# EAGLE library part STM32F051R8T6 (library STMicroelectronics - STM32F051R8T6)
Source: Datasheet
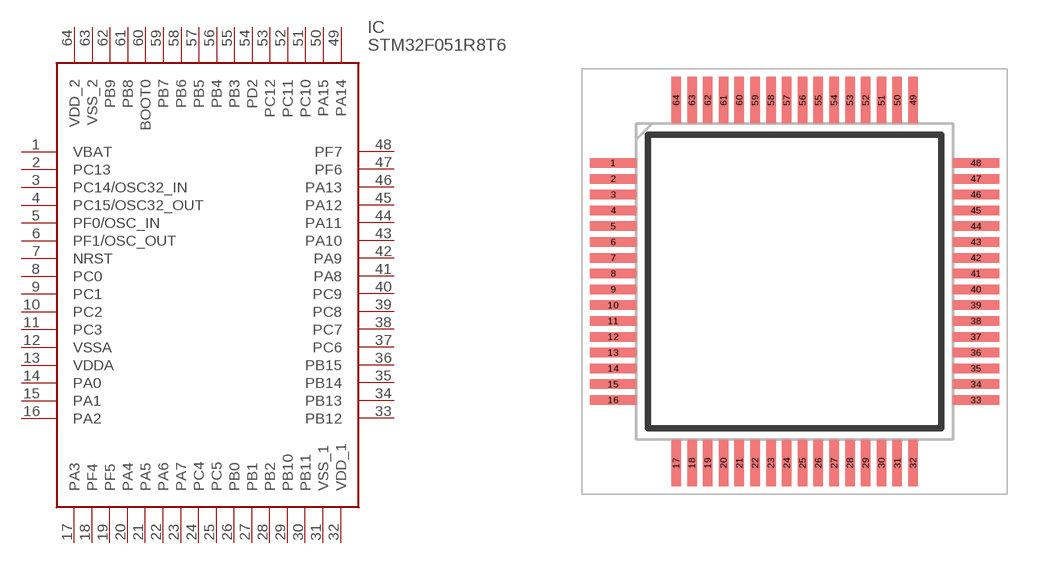
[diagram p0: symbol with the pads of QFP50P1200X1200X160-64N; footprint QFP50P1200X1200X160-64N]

Designator prefix IC

## STM32F051R8T6 (ALLIED_NUMBER: 70390941; ALLIED_PRICE-STOCK: http://www.alliedelec.com/stmicroelectronics-stm32f051r8t6/70390941/; HEIGHT: 1.6mm; MANUFACTURER_NAME: STMicroelectronics; MANUFACTURER_PART_NUMBER: STM32F051R8T6; MOUSER_PART_NUMBER: 511-STM32F051R8T6; MOUSER_PRICE-STOCK: https://www.mouser.com/Search/Refine.aspx?Keyword=511-STM32F051R8T6; RS_PART_NUMBER: 7618683P; RS_PRICE-STOCK: http://uk.rs-online.com/web/p/products/7618683P)  [QFP50P1200X1200X160-64N]
1  VBAT
2  PC13
3  PC14/OSC32_IN  in
4  PC15/OSC32_OUT  out
5  PF0/OSC_IN  in
6  PF1/OSC_OUT  out
7  NRST  in
8  PC0
9  PC1
10  PC2
11  PC3
12  VSSA  pwr
13  VDDA  pwr
14  PA0
15  PA1
16  PA2
17  PA3
18  PF4
19  PF5
20  PA4
21  PA5
22  PA6
23  PA7
24  PC4
25  PC5
26  PB0
27  PB1
28  PB2
29  PB10
30  PB11
31  VSS_1  pwr
32  VDD_1  pwr
33  PB12
34  PB13
35  PB14
36  PB15
37  PC6
38  PC7
39  PC8
40  PC9
41  PA8
42  PA9
43  PA10
44  PA11
45  PA12
46  PA13
47  PF6
48  PF7
49  PA14
50  PA15
51  PC10
52  PC11
53  PC12
54  PD2
55  PB3
56  PB4
57  PB5
58  PB6
59  PB7
60  BOOT0
61  PB8
62  PB9
63  VSS_2  pwr
64  VDD_2  pwr

## Footprint QFP50P1200X1200X160-64N (pad centres in mm)
LQFP64-10 x 10 mm 64 pin
smd 1.475 x 0.3: 1 -5.738,3.75; 2 -5.738,3.25; 3 -5.738,2.75; 4 -5.738,2.25; 5 -5.738,1.75; 6 -5.738,1.25; 7 -5.738,0.75; 8 -5.738,0.25; 9 -5.738,-0.25; 10 -5.738,-0.75; 11 -5.738,-1.25; 12 -5.738,-1.75; 13 -5.738,-2.25; 14 -5.738,-2.75; 15 -5.738,-3.25; 16 -5.738,-3.75; 33 5.738,-3.75; 34 5.738,-3.25; 35 5.738,-2.75; 36 5.738,-2.25; 37 5.738,-1.75; 38 5.738,-1.25; 39 5.738,-0.75; 40 5.738,-0.25; 41 5.738,0.25; 42 5.738,0.75; 43 5.738,1.25; 44 5.738,1.75; 45 5.738,2.25; 46 5.738,2.75; 47 5.738,3.25; 48 5.738,3.75
smd 0.3 x 1.475: 17 -3.75,-5.738; 18 -3.25,-5.738; 19 -2.75,-5.738; 20 -2.25,-5.738; 21 -1.75,-5.738; 22 -1.25,-5.738; 23 -0.75,-5.738; 24 -0.25,-5.738; 25 0.25,-5.738; 26 0.75,-5.738; 27 1.25,-5.738; 28 1.75,-5.738; 29 2.25,-5.738; 30 2.75,-5.738; 31 3.25,-5.738; 32 3.75,-5.738; 49 3.75,5.738; 50 3.25,5.738; 51 2.75,5.738; 52 2.25,5.738; 53 1.75,5.738; 54 1.25,5.738; 55 0.75,5.738; 56 0.25,5.738; 57 -0.25,5.738; 58 -0.75,5.738; 59 -1.25,5.738; 60 -1.75,5.738; 61 -2.25,5.738; 62 -2.75,5.738; 63 -3.25,5.738; 64 -3.75,5.738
